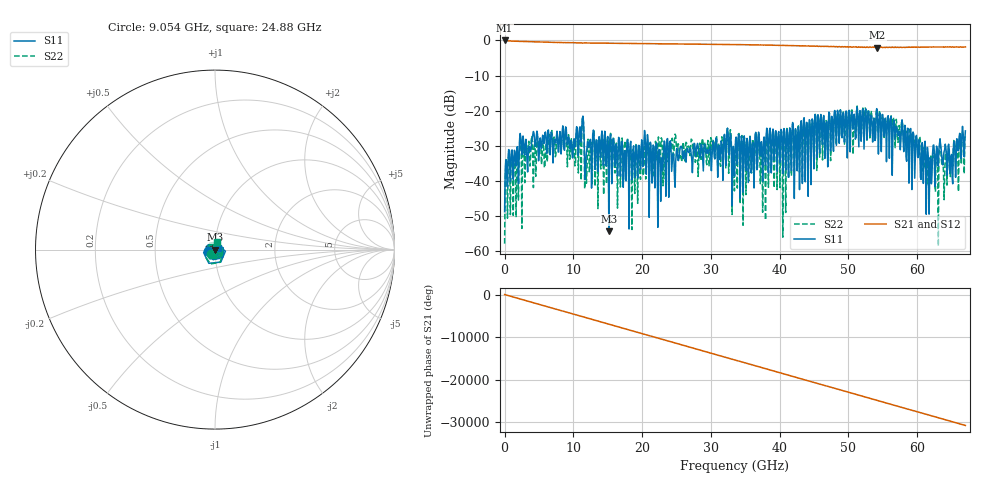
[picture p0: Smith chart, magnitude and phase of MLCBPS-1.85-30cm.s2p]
!China Electronics Technology Instruments Limited Company,3672E,ZFL00052,2.0.3
!Calibration ON : 2P/1,2
!S2P File: Measurements: S11, S21, S12, S22: lin Frequency Sweep
!Thursday, April 15, 2021  13 : 54
# Hz  S  dB  R 50.000
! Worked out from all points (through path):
!   801 points, 10 MHz to 67 GHz, reference 50 ohm
!   highest |S21| = -0.03 dB at 10 MHz (marker M1); lowest = -2.1 dB at 54.19 GHz (marker M2)
!   lowest |S11| = -54.3 dB at 15.17 GHz (marker M3), VSWR 1.00, Z = 49.8 - j0.0248 ohm
!   |S11| at or under -10 dB: start of sweep to end of sweep
!   |S22| runs from -58.5 to -18.7 dB; largest |S21 - S12| = 0.011
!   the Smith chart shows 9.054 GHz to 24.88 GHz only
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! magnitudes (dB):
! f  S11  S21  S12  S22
! 10 MHz  -48.7  0.0  0.0  -57.8
! 428.7 MHz  -41.7  -0.1  -0.1  -50.6
! 2.103 GHz  -34.1  -0.3  -0.3  -35.6
! 9.807 GHz  -31.2  -0.7  -0.7  -30.3
! 11.23 GHz  -24.6  -0.7  -0.7  -26.3
! 11.98 GHz  -30.7  -0.7  -0.7  -37.0
! 15.17 GHz  -54.3  -0.8  -0.8  -39.3
! 17.68 GHz  -40.0  -0.9  -0.9  -33.8
! 18.68 GHz  -31.1  -0.9  -0.9  -31.1
! 20.61 GHz  -38.1  -0.9  -0.9  -34.1
! 22.37 GHz  -33.9  -1.0  -1.0  -27.5
! 32.58 GHz  -31.8  -1.2  -1.2  -37.8
! 33.51 GHz  -32.4  -1.2  -1.2  -34.1
! 36.77 GHz  -35.8  -1.3  -1.3  -36.2
! 37.61 GHz  -30.8  -1.3  -1.3  -34.4
! 44.73 GHz  -22.3  -1.6  -1.6  -22.5
! 54.19 GHz  -20.1  -2.1  -2.1  -20.0
! 55.86 GHz  -25.7  -2.0  -2.0  -24.5
! 60.13 GHz  -33.3  -1.9  -1.9  -30.6
! 61.64 GHz  -34.1  -1.9  -1.9  -36.7
! 62.81 GHz  -30.1  -1.9  -1.9  -31.6
! 67 GHz  -25.7  -1.9  -1.9  -27.3
